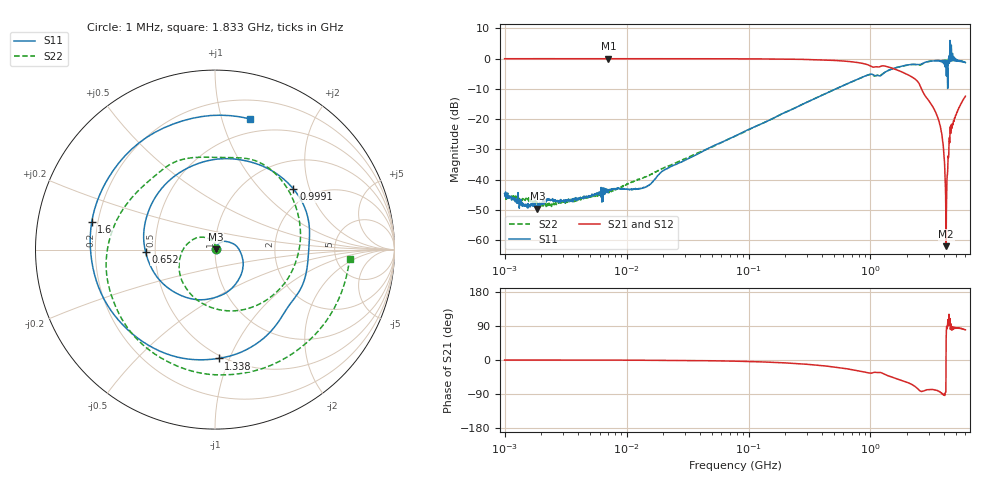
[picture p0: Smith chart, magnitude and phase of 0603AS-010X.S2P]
!s-Parameter Generated by FASTRON Sdn. Bhd.
!FASTRON P/N : 0603AS-010X
!Keysight Technologies: E5071C_MY46733604_B.14.02
!Date: Tue Oct 10 11:30:13 2023
!Version  :Rev01  Tue Oct 10 11:30:13 2023
!Data & Calibration Information:
!Freq  S11:SOLT2(ON)  S21:SOLT2(ON)  S12:SOLT2(ON)  S22:SOLT2(ON)
!PortZ  Port1:50+j0  Port2:50+j0
!When reading reference impedance value at option line is always used.
! Remarks : This data is being provided solely for informational purposes.
# Hz S dB R 50
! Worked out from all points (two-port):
!   1601 points, 1 MHz to 6 GHz, reference 50 ohm
!   highest |S21| = -0.03 dB at 7.106 MHz (marker M1); lowest = -62.0 dB at 4.171 GHz (marker M2)
!   |S21| within 3 dB of the highest: start of sweep to 1.472 GHz
!   lowest |S11| = -49.6 dB at 1.855 MHz (marker M3), VSWR 1.01, Z = 50.3 + j0.13 ohm
!   |S11| at or under -10 dB: start of sweep to 521.4 MHz
!   |S22| runs from -48.9 to -0.5 dB; largest |S21 - S12| = 0.0055
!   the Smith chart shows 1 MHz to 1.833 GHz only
!   S11 on the Smith chart (normalised r, x): 1 MHz: 1.01, +0.00; 652 MHz: 0.44, -0.01; 999.1 MHz: 1.61, +1.57; 1.338 GHz: 0.48, -0.91; 1.6 GHz: 0.18, +0.11; 1.833 GHz: 0.37, +1.24
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1000000  -44.63 13.8  -0.05 -0.0  -0.04 0.0  -45.23 13.9
1855321  -49.59 23.0  -0.04 -0.1  -0.04 -0.1  -47.77 12.3
4277066  -46.10 36.3  -0.05 -0.2  -0.04 -0.2  -46.06 48.5
7105645  -43.46 45.8  -0.03 -0.4  -0.05 -0.3  -43.84 60.5
1.823719e7  -38.46 64.6  -0.04 -0.8  -0.05 -0.7  -36.93 74.7
7.757876e7  -25.61 50.7  -0.08 -3.1  -0.08 -3.1  -25.67 107.7
3.307917e8  -13.64 -48.3  -0.33 -12.4  -0.33 -12.3  -13.65 -162.8
6.519555e8  -8.25 -177.9  -0.93 -23.6  -0.94 -23.5  -8.25 -54.0
9.990907e8  -5.16 37.8  -2.44 -34.7  -2.44 -34.6  -5.27 59.1
1.337692e9  -4.34 -88.1  -2.56 -39.4  -2.56 -39.2  -4.33 -175.4
1.414819e9  -3.82 -118.8  -2.83 -42.4  -2.83 -42.3  -3.88 -148.7
1.599924e9  -3.05 167.3  -3.55 -48.2  -3.55 -48.2  -3.09 -85.0
1.833007e9  -2.45 75.0  -4.53 -54.7  -4.53 -54.7  -2.48 -4.1
2.24757e9  -1.89 -87.9  -6.38 -66.9  -6.39 -66.8  -1.98 141.2
2.760696e9  -1.37 78.0  -11.85 -81.2  -11.84 -81.2  -1.46 -30.3
3.17898e9  -0.79 -84.6  -15.42 -77.8  -15.41 -77.8  -0.78 118.3
3.604213e9  -0.68 112.0  -20.15 -81.6  -20.15 -81.7  -0.61 -89.6
3.867453e9  -1.26 8.3  -25.83 -90.0  -25.82 -90.2  -0.68 5.6
4.171191e9  -4.43 -102.5  -61.99 52.6  -61.98 54.5  -0.60 116.3
4.573027e9  2.23 103.4  -23.39 95.4  -23.37 95.2  -0.60 -97.0
5.356463e9  -0.77 173.6  -16.09 84.0  -16.09 84.1  -0.77 -169.6
6e9  -1.35 -67.2  -12.45 79.8  -12.44 80.0  -1.13 66.7
